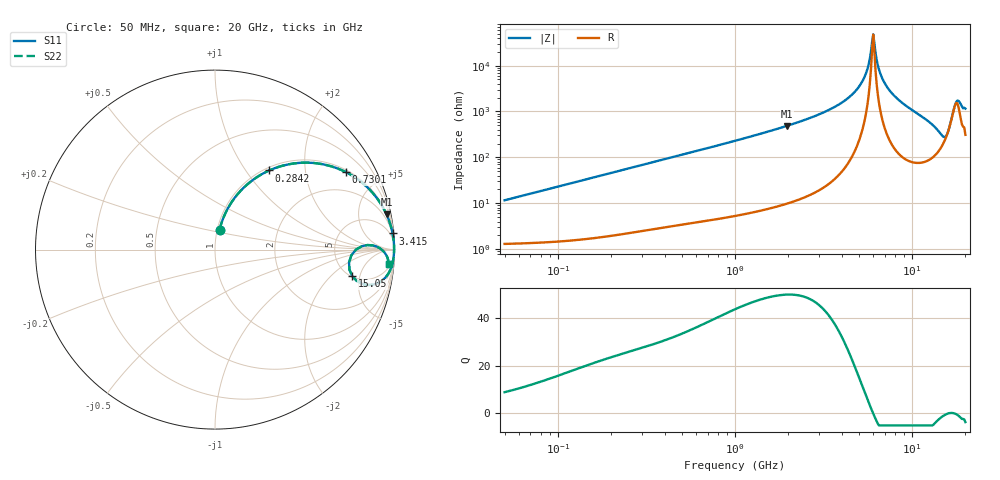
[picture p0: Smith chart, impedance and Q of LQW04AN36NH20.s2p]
!Murata Part Number: LQW04AN36NH20
!These Parameters are Measured in Series Mode Connection
!  o--[Z]--o
!Port1  Port2
!  o-------o
!Freq. Start=50[MHz] Stop=20[GHz], 401[Steps]
# Hz S RI R 50
!Freq.(Hz) S11(Real) S11(Imag) S21(Real) S21(Imag) S12(Real) S12(Imag) S22(Real) S22(Imag)
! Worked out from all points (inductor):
!   401 points, 50 MHz to 20 GHz, reference 50 ohm
!   read as one part in series: L = 36.7 nH near 51.52 MHz
!   highest Q = 49.6 at 1.962 GHz (marker M1), where L = 39.4 nH
!   self-resonance near 5.944 GHz
!   S11 on the Smith chart (normalised r, x): 50 MHz: 1.03, +0.23; 284.2 MHz: 1.05, +1.30; 730.1 MHz: 1.09, +3.32; 3.415 GHz: 2, +22; 15.05 GHz: 5.10, -3.83; 20 GHz: 7, -22
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5e7  0.0255 0.111  0.9745 -0.111  0.9745 -0.111  0.0255 0.111
1.364002e8  0.1013 0.2769  0.8987 -0.2769  0.8987 -0.2769  0.1013 0.2769
2.841629e8  0.3025 0.4411  0.6975 -0.4411  0.6975 -0.4411  0.3025 0.4411
3.721004e8  0.4199 0.477  0.5801 -0.477  0.5801 -0.477  0.4199 0.477
7.30116e8  0.7287 0.4319  0.2713 -0.4319  0.2713 -0.4319  0.7287 0.4319
1e9  0.8348 0.36  0.1652 -0.36  0.1652 -0.36  0.8348 0.36
1.962148e9  0.9556 0.1961  0.0444 -0.1961  0.0444 -0.1961  0.9556 0.1961
2.728004e9  0.98 0.1297  0.02 -0.1297  0.02 -0.1297  0.98 0.1297
3.415248e9  0.9896 0.0899  0.0104 -0.0899  0.0104 -0.0899  0.9896 0.0899
4.34015e9  0.9955 0.051  0.00454 -0.051  0.00454 -0.051  0.9955 0.051
5.041459e9  0.9973 0.0277  0.00267 -0.0277  0.00267 -0.0277  0.9973 0.0277
5.515528e9  0.9978 0.0138  0.00215 -0.0138  0.00215 -0.0138  0.9978 0.0138
5.856089e9  0.9979 0.00457  0.00206 -0.00457  0.00206 -0.00457  0.9979 0.00457
6.034176e9  0.9979 -9.73e-05  0.00209 9.73e-05  0.00209 9.73e-05  0.9979 -9.73e-05
6.125241e9  0.9979 -0.00244  0.00212 0.00244  0.00212 0.00244  0.9979 -0.00244
6.601595e9  0.9975 -0.0143  0.00251 0.0143  0.00251 0.0143  0.9975 -0.0143
7.442007e9  0.996 -0.0339  0.00397 0.0339  0.00397 0.0339  0.996 -0.0339
1.238412e10  0.9528 -0.1518  0.0472 0.1518  0.0472 0.1518  0.9528 -0.1518
1.504638e10  0.7648 -0.1475  0.2352 0.1475  0.2352 0.1475  0.7648 -0.1475
1.597544e10  0.7858 3.84e-05  0.2142 -3.84e-05  0.2142 -3.84e-05  0.7858 3.84e-05
1.774144e10  0.9431 -0.0148  0.0569 0.0148  0.0569 0.0148  0.9431 -0.0148
2e10  0.9709 -0.079  0.0291 0.079  0.0291 0.079  0.9709 -0.079
